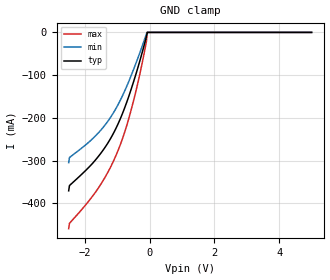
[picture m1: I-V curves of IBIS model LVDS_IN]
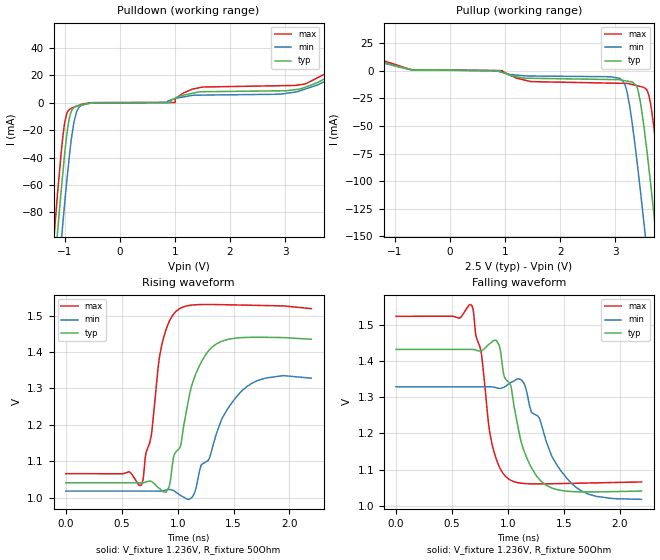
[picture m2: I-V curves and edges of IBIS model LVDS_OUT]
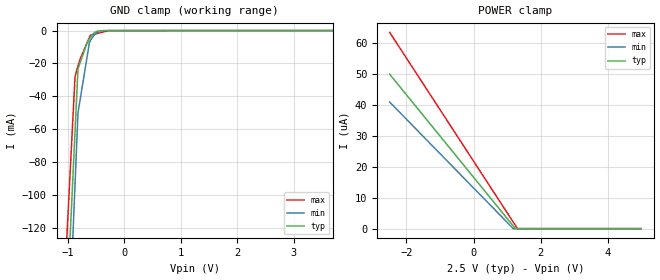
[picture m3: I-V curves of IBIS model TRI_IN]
| Texas Instruments Incorporated
| 2:12 Low Additive Jitter LVDS buffer
| Marketing part#   Voltage Range   Package-type   #pins/pkg drawing
| CDCLVD1212   2.375V-3.625V   QFN   40-pin QFN
[IBIS Ver]   4.0
[File name]   cdclvd1212.ibs
[File Rev]   1.2
[Date]   10/23/2018
[Source]   spectre simulations
   Texas Instruments Incorporated.
   Analog eLab Design Center, HPA
   12500 TI Blvd
   Dallas, TX -75243
   For Support e-mail: elab_scm_ibis@list.ti.com
[Notes]   Revision History:
   Rev 1.2: 10/23/2018
   - TRI_IN model updated to reflect true electrical behavior.
   - VBB_OUT model removed  due  to inaccurary in describing
   termination behavior.
   Rev 1.1: 8/29/2013
   - Updated LVDS_IN to correct POWER and GROUND Clamp models.
   Rev 1.0: 07/06/2010
   - C_comp although listed in numberical order of value are obtained from varying PVT conditions.
   For PVT conditions for eachspecific value, refer to the buffer description under repective [Model].
   IBIS model user is responsible for using appropriate C_comp to simulate for Signal Integrity.
   - TISPice simulation of Clamp current does not match silicon
   - POWER and GND clamp for TRI_IN, D_REB_IN non-monotonic due circuit design
   - GND clamp for LVDS_IN non-monotonic due to circuit design
   - LVDS_OUT pullup/pulldown non-monotonic as a result of circuit design
[Disclaimer] This model is designed as an aid for customers of Texas Instruments.
 TI and its licensors and suppliers make no warranties, either expressed
 or implied, with respect to this  model, including the warranties of
 merchantability or fitness for a particular purpose.
 The model is provided solely on an "as is" basis. The entire risk as to
 its quality and performance is with the customer.
[Copyright] (C)Copyright 2013 Texas Instruments Incorporated.
   All rights reserved.
|   Component CDCLVD1212
[Component]   CDCLVD1212
[Manufacturer]  Texas Instruments Incorporated
[Package]   |QFN (RHA) 40-pin
|   typ   min   max
R_pkg   0.0658   0.0248   0.0806
L_pkg   0.8404nH   0.6985nH   1.0659nH
C_pkg   0.1111pF   0.1026pF   0.1480pF
[Pin]   signal_name   model_name   R_pin   L_pin   C_pin
1   IN_SEL   TRI_IN   0.02222  0.62828n  0.38909p
2   INP1   LVDS_IN   0.17239  2.51308n  0.20075p
3   INN1   LVDS_IN   0.15946  2.30909n  0.18422p
4   VAC_REF1   NC   0.15034  2.16565n  0.17563p
5   VCC   POWER   0.07337  1.60844n  0.22970p
6   VCC   POWER   0.14583  2.09475n  0.17007p
7   VAC_REF0   NC   0.15034  2.16566n  0.17301p
8   INN0   LVDS_IN   0.15946  2.30910n  0.18375p
9   INP0   LVDS_IN   0.17239  2.51309n  0.19137p
10   NC   NC   0.00063  0.06887n  0.02810p
11   VCC   POWER   0.18416  2.69986n  0.19951p
12   OUTP0   LVDS_OUT   0.16882  2.45528n  0.19506p
13   OUTN0   LVDS_OUT   0.15676  2.26409n  0.18051p
14   OUTP1   LVDS_OUT   0.14873  2.13665n  0.17088p
15   OUTN1   LVDS_OUT   0.14547  2.08444n  0.16699p
16   OUTP2   LVDS_OUT   0.14735  2.11295n  0.16908p
17   OUTN2   LVDS_OUT   0.15415  2.21906n  0.17693p
18   OUTP3   LVDS_OUT   0.16521  2.39250n  0.18972p
19   OUTN3   LVDS_OUT   0.17965  2.62009n  0.20065p
20   VCC   POWER   0.09374  2.30558n  0.25381p
21   GND   GND   0.09097  2.18287n  0.25251p
22   OUTP4   LVDS_OUT   0.17359  2.52348n  0.19352p
23   OUTN4   LVDS_OUT   0.16039  2.31449n  0.18384p
24   OUTP5   LVDS_OUT   0.15092  2.16505n  0.17293p
25   OUTN5   LVDS_OUT   0.14601  2.08754n  0.16610p
26   OUTP6   LVDS_OUT   0.14601  2.08755n  0.16609p
27   OUTN6   LVDS_OUT   0.15092  2.16506n  0.17293p
28   OUTP7   LVDS_OUT   0.16039  2.31450n  0.18384p
29   OUTN7   LVDS_OUT   0.17359  2.52349n  0.19352p
30   GND   GND   0.09097  2.18287n  0.25251p
31   VCC   POWER   0.09374  2.30558n  0.25381p
32   OUTP8   LVDS_OUT   0.17965  2.62008n  0.20065p
33   OUTN8   LVDS_OUT   0.16521  2.39249n  0.18972p
34   OUTP9   LVDS_OUT   0.15415  2.21905n  0.17694p
35   OUTN9   LVDS_OUT   0.14735  2.11294n  0.16909p
36   OUTP10   LVDS_OUT   0.14547  2.08445n  0.16699p
37   OUTN10   LVDS_OUT   0.14873  2.13666n  0.17088p
38   OUTP11   LVDS_OUT   0.15676  2.26410n  0.18053p
39   OUTN11   LVDS_OUT   0.16882  2.45529n  0.19523p
40   VCC   POWER   0.18416  2.69987n  0.20183p
[Diff_pin]   inv_pin   vdiff   tdelay_typ   tdelay_min   tdelay_max
| The 'OUTPx' pin is Diff_pin and the 'OUTNx' pin is the inv_pin
| The 'INPx' pin is Diff_pin and the 'INNx' pin is the inv_pin
2   3   0.200   0 0 0
8   9   0.200   0 0 0
12   13   0.200   0 0 0
14   15   0.200   0 0 0
16   17   0.200   0 0 0
18   19   0.200   0 0 0
22   23   0.200   0 0 0
24   25   0.200   0 0 0
26   27   0.200   0 0 0
28   29   0.200   0 0 0
32   33   0.200   0 0 0
34   35   0.200   0 0 0
36   37   0.200   0 0 0
38   39   0.200   0 0 0
| Models and submodels in the file (3): LVDS_IN (Input), LVDS_OUT (Output), TRI_IN (Input)
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|   LVDS Input Model
[Model]   LVDS_IN
Model_type   Input
|Signals   INP0,INN0,INP1,INN1
Vinh = 1.6
Vinl = 0.3
| variable   typ   min   max
|   (nom PVT)   (slow PVT)   (fast PVT)
C_comp   3.121pF   2.849pF   3.193pF
| Ccomp comes from PVT, calculated at 800MHz.
| Nom PVT is nom process, 2.5V, 25C
| slow PVT is weak process, 2.375V, 105C
| Fast process is strong process, 2.625V, -40C
|   typ   min   max
[Voltage Range]   2.5   2.375   2.625
[Temperature Range]   25   105   -40
[Power Clamp Reference]   2.5   2.375   2.625
[GND Clamp Reference]   0   0   0
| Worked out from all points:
|   GND clamp passes 1 mA (typ) near -0.08 V on its own axis
[GND Clamp]
|   Voltage   I(typ)   I(min)   I(max)
-2.5V     -370.8mA   -304.9mA   -459.4mA
-2.475V   -358.5mA   -293mA     -446.8mA
-1.9V     -317.5mA   -258.4mA   -396.7mA
-1.5V     -282.1mA   -228.1mA   -354.5mA
-1.225V   -250.8mA   -200.9mA   -318mA
-975mV    -214.1mA   -169mA     -276.3mA
-700mV    -161.8mA   -124.9mA   -216.1mA
-450mV    -104.2mA   -77.57mA   -145.7mA
-150mV    -24.38mA   -14.67mA   -41.36mA
-100mV    -9.871mA   -3.55mA    -21.64mA
-75.01mV  0A         0A         0A
5V        0A         0A         0A
[POWER Clamp]
|   Voltage   I(typ)   I(min)   I(max)
-2.5V     0A         0A         0A
-2.475V   0A         0A         0A
-2.45V    0A         0A         0A
5V        0A         0A         0A
|   LVDS_OUT Model
[Model]   LVDS_OUT
Model_type   Output
| Signals   OUTP0,OUTN0,OUTP1,OUTN1,OUTP2,OUTN2,OUTP3,OUTN3,OUTP4,OUTN4,OUTP5,OUTN5
|   OUTP6,OUTN6,OUTP7,OUTN7,OUTP8,OUTN8,OUTP9,OUTN9,OUTP10,OUTN10,OUTP11,OUTN11
Polarity   Non-Inverting
Vmeas = 1.25
Vref = 1.25
Cref = 15pF
Rref = 50
| variable   typ   min   max
|   (nom PVT)   (slow PVT)   (fast PVT)
C_comp   1.275pF   1.175pF   1.317pF
| Ccomp comes from PVT corner simulations
| Nom PVT is nom process, 2.5V, 25C
| slow PVT is weak process, 2.375V, 105C
| Fast process is strong process, 2.625V, -40C
[Voltage Range]   2.5   2.375   2.625
[Temperature Range]   25   105   -40
[Pullup Reference]   2.5   2.375   2.625
[Pulldown Reference]   0   0   0
[Power Clamp Reference]   2.5   2.375   2.625
[GND Clamp Reference]   0   0   0
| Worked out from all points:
|   slope of the pulldown table from 0 to 0.375 V, typ, clamps not added: 11.9 kohm
|   slope of the pullup table from 0 to 0.375 V, typ, clamps not added: 2.06 kohm
|   falling waveform, V_fixture 1.236V, R_fixture 50Ohm: 20-80 % time 216ps typ, 313ps min, 114ps max; typ from 1.43 V to 1.04 V
|   rising waveform, V_fixture 1.236V, R_fixture 50Ohm: 20-80 % time 213ps typ, 297ps min, 111ps max; typ from 1.04 V to 1.44 V
[Pulldown]
|   Voltage   I(typ)   I(min)   I(max)
-2.5V     -819.9mA   -841.2mA   -808.9mA
-1.205V   -132.7mA   -170.8mA   -104.8mA
-1.179V   -119.9mA   -157.8mA   -91.4mA
-1.126V   -94.38mA   -132.6mA   -65.81mA
-1.057V   -62.54mA   -100.1mA   -34.83mA
-992.5mV  -35.05mA   -71.07mA   -13.52mA
-904.2mV  -9.792mA   -35.76mA   -4.869mA
-801.5mV  -2.839mA   -9.874mA   -2.967mA
-497.6mV  -107.4uA   -219.6uA   -77.81uA
1.006V    3.123mA    2.958mA    13.07uA
3.348V    10.9mA     9.549mA    13.39mA
4.992V    48.76mA    47.89mA    54.44mA
[Pullup]
|   Voltage   I(typ)   I(min)   I(max)
-2.5V     34.99mA    35.32mA    37.69mA
-673.6mV  752.9uA    742.8uA    631.1uA
3.09V     -8.286mA   -7.075mA   -11.46mA
3.202V    -9.311mA   -16.77mA   -11.57mA
3.31V     -10.29mA   -48.27mA   -12.56mA
3.416V    -18.21mA   -90.66mA   -13.83mA
3.525V    -51.64mA   -139.2mA   -15.42mA
3.637V    -99.27mA   -190.6mA   -28.34mA
3.71V     -133.1mA   -225.4mA   -54.42mA
3.766V    -159.3mA   -252.7mA   -79.01mA
3.928V    -237.8mA   -331.5mA   -155.2mA
4.992V    -776.9mA   -866.8mA   -698.2mA
[Ramp]
R_load = 50
|   typ   min   max
dV/dt_r   0.238696/2.15967e-10   0.19168/3.14155e-10   0.275901/1.13765e-10
dV/dt_f   0.234348/2.15967e-10   0.186163/3.14155e-10   0.274079/1.13765e-10
[Falling Waveform]
V_fixture = 1.236V
V_fixture_min = 1.173V
V_fixture_max = 1.294V
R_fixture = 50Ohm
C_fixture = 0F
|   Time   V(typ)   V(min)   V(max)
0s        1.431V     1.328V     1.523V
675ps     1.432V     1.328V     1.553V
765ps     1.428V     1.328V     1.417V
855ps     1.451V     1.328V     1.176V
920ps     1.445V     1.324V     1.11V
1.01ns    1.34V      1.337V     1.073V
1.135ns   1.16V      1.342V     1.062V
1.305ns   1.066V     1.219V     1.061V
1.62ns    1.039V     1.049V     1.062V
2.195ns   1.041V     1.018V     1.066V
[Rising Waveform]
V_fixture = 1.236V
V_fixture_min = 1.173V
V_fixture_max = 1.294V
R_fixture = 50Ohm
C_fixture = 0F
|   Time   V(typ)   V(min)   V(max)
0s        1.041V     1.018V     1.066V
675ps     1.04V      1.018V     1.035V
765ps     1.044V     1.018V     1.172V
855ps     1.021V     1.018V     1.415V
920ps     1.027V     1.022V     1.481V
1.01ns    1.133V     1.009V     1.518V
1.135ns   1.317V     1.004V     1.53V
1.305ns   1.413V     1.13V      1.531V
1.62ns    1.44V      1.306V     1.529V
2.195ns   1.435V     1.328V     1.52V
|   TRI_IN Input Model
[Model]   TRI_IN
Model_type   Input
Vinl = 0.475
Vinh = 1.8375
|   typ   min   max
C_comp   1.974pF   1.947pF   1.983pF
[Voltage Range]   2.5   2.375   2.625
[Temperature Range]   25   105   -40
[Power Clamp Reference]   2.5   2.375   2.625
[GND Clamp Reference]   0   0   0
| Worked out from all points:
|   GND clamp passes 1 mA (typ) near -0.51 V on its own axis
[GND Clamp]
|   Voltage   I(typ)   I(min)   I(max)
-2.5V     -1.519A    -1.599A    -1.46A
-1.383V   -435.2mA   -519.8mA   -372mA
-872mV    -61.4mA    -93.54mA   -27.86mA
-820mV    -23.3mA    -50.1mA    -21.6mA
-782.5mV  -19.62mA   -42.18mA   -17.41mA
-670mV    -8.564mA   -18.42mA   -8.334mA
-617.5mV  -5.055mA   -7.338mA   -4.098mA
-602.5mV  -4.217mA   -6.329mA   -2.888mA
-497.5mV  -686.1uA   -1.614mA   -1.968mA
-415mV    -96.99uA   -336uA     -1.246mA
-275.7mV  -21.08uA   -26.56uA   -26.45uA
5V        0A         0A         0A
[POWER Clamp]
|   Voltage   I(typ)   I(min)   I(max)
-2.5V     49.93uA    40.92uA    63.45uA
1.183V    882.3nA    41.92nA    2.147uA
1.242V    83.42nA    0A         1.149uA
1.31V     0A         0A         25.11nA
5V        0A         0A         0A
